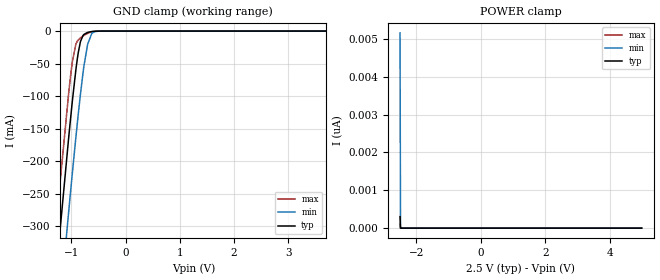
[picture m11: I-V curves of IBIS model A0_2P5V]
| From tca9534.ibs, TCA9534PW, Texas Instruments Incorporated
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[Model]   A0_2P5V
Model_type   Input
Vinl = .8
Vinh = 2
|   typ   min   max
|   (nom PVT)   (slow PVT)   (fast PVT)
C_comp   1.373p   1.325p   1.458p
| Where   nom PVT is  Nominal Process, 2.5V, 27C
|   Fast PVT is Strong Process, 2.75V, -40C
|   Slow PVT is Weak Process, 2.25V, 125C
[Voltage Range]   2.5   2.25   2.75
[Temperature Range]   27   125   -40
[Power Clamp Reference]   2.5   2.25   2.75
[GND Clamp Reference]   -0   -0   -0
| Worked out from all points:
|   GND clamp passes 1 mA (typ) near -0.64 V on its own axis
[GND Clamp]
|   Voltage   I(typ)   I(min)   I(max)
-2.5V     -1.556A    -1.668A    -1.487A
-1.48V    -562.8mA   -678.5mA   -490.3mA
-1.27V    -364.2mA   -480.4mA   -291.4mA
-1.218V   -315.6mA   -431.6mA   -242.9mA
-1.052V   -167.5mA   -281.4mA   -98.76mA
-977.5mV  -105.3mA   -215.6mA   -45.46mA
-917.5mV  -60.82mA   -164.9mA   -20.67mA
-835mV    -17.55mA   -99.86mA   -10.75mA
-700mV    -2.035mA   -20.56mA   -3.474mA
-625mV    -707.9uA   -4.145mA   -1.242mA
-490mV    -59.3uA    -153.7uA   -79.31uA
4.992V    0A         0A         0A
[POWER Clamp]
|   Voltage   I(typ)   I(min)   I(max)
-2.5V     306.4pA    5.157nA    106.3pA
-2.485V   0A         0A         0A
-2.478V   0A         0A         0A
4.992V    0A         0A         0A
